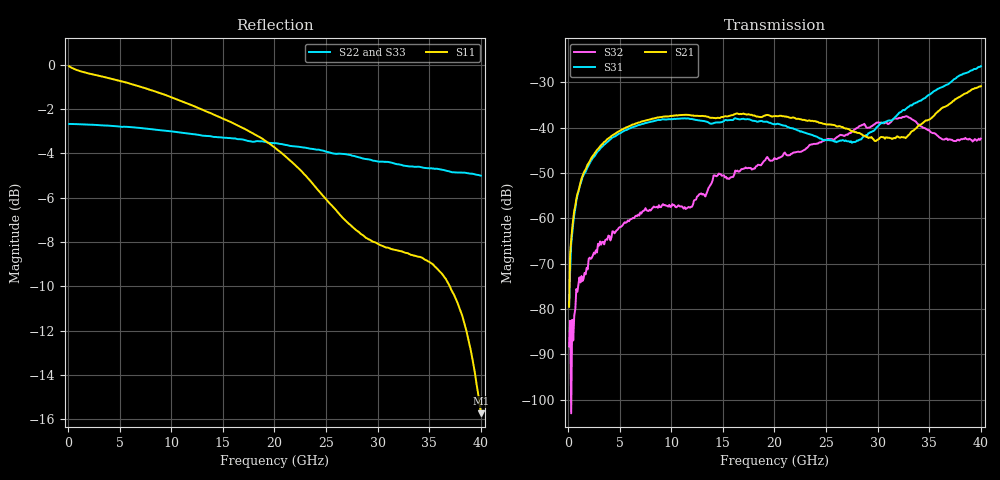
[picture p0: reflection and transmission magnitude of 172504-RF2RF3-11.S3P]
!  3-Port S-parameters saved by WinCal
! VAR MeasName=S-Parameters (CALIBRATED_DATA) read from VNA (N5245A)
! VAR MeasDate=2017-3-15 11:04:11
! VAR NAME=172504-RF2RF3-11
! VAR FILENAME=172504-RF2RF3-11.S3P
! VAR DATE=2017-3-15 11:04:11
! VAR PHYS_PORTS=1,2,3
# Hz S DB R 50
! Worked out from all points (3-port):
!   400 points, 100 MHz to 40 GHz, reference 50 ohm
!   strongest paths, dB at 100 MHz, 10.1 GHz, 20.1 GHz, 30.1 GHz, 40 GHz:
!     S21: -79.5, -37.4, -37.4, -42.5, -30.8
!     S31: -79.3, -38.1, -39.3, -39.5, -26.4
!     S32: -88.2, -56.9, -46.9, -38.8, -42.4
!   lowest |S11| = -15.7 dB at 40 GHz (marker M1), VSWR 1.39, Z = 37.5 - j6.95 ohm
!   |S11| at or under -10 dB: 36.99 GHz to end of sweep
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1e8  -0.06 -1.8  -74.38 77.4  -78.35 105.8
     -79.50 79.1  -2.67 179.8  -87.56 -151.4
     -79.29 97.5  -88.23 134.3  -2.63 179.8
2e8  -0.10 -3.4  -67.38 100.3  -71.30 102.7
     -67.78 99.3  -2.67 179.5  -88.13 28.4
     -71.56 114.8  -82.57 -62.4  -2.64 179.6
9e8  -0.24 -13.5  -54.58 86.9  -55.29 89.9
     -54.62 87.0  -2.68 178.0  -77.41 86.5
     -55.02 90.8  -76.19 98.0  -2.65 178.1
3.5e9  -0.55 -48.3  -43.21 57.0  -43.79 57.2
       -43.13 56.8  -2.74 172.5  -65.32 83.2
       -43.72 57.5  -65.73 80.4  -2.70 172.8
1.19e10  -1.81 -137.1  -37.25 -14.6  -38.07 -14.6
         -37.27 -14.6  -3.12 155.2  -57.58 71.0
         -38.08 -14.6  -57.46 71.7  -3.05 156.1
2.01e10  -3.76 149.5  -37.45 -59.7  -39.13 -56.7
         -37.42 -59.0  -3.54 137.6  -46.69 40.5
         -39.25 -56.2  -46.86 38.5  -3.47 138.5
2.47e10  -5.91 93.2  -39.10 -87.1  -42.58 -67.8
         -39.11 -86.5  -3.87 126.1  -42.83 16.3
         -42.79 -67.8  -42.88 15.9  -3.86 127.1
2.96e10  -8.00 14.7  -42.34 -100.2  -40.35 -44.9
         -42.57 -99.0  -4.33 113.4  -39.35 -27.2
         -40.73 -44.1  -39.33 -27.2  -4.31 114.0
3.53e10  -8.99 -69.2  -37.34 -80.8  -31.86 -69.4
         -37.68 -78.7  -4.69 97.3  -41.22 -110.3
         -32.25 -66.4  -41.18 -109.8  -4.89 97.9
4e10  -15.74 -146.5  -30.53 -119.9  -26.26 -116.8
      -30.82 -116.9  -5.00 81.5  -42.45 -140.1
      -26.42 -112.4  -42.41 -137.2  -5.25 82.5
